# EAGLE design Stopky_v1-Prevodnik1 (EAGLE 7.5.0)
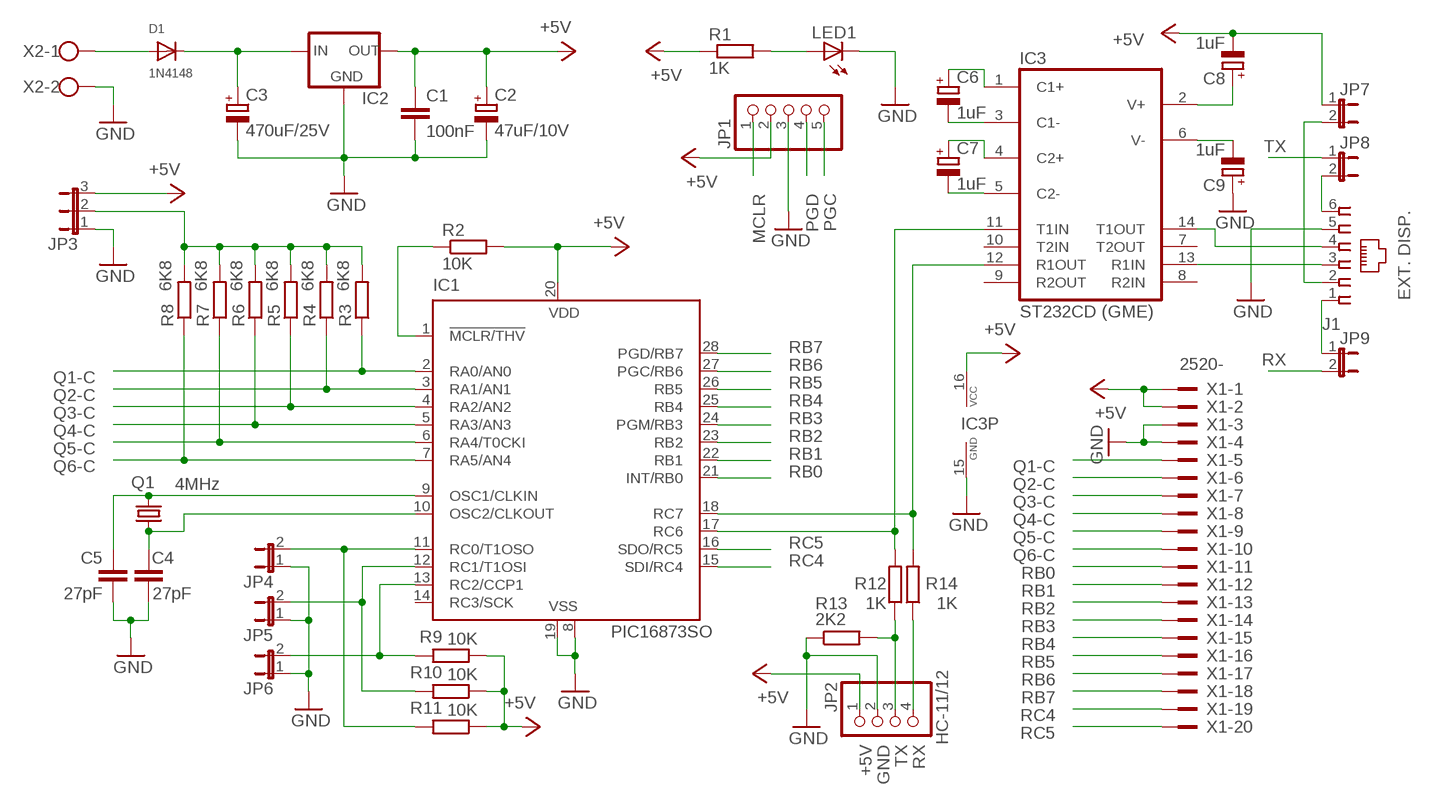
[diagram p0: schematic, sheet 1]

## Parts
C1  100nF  C-EUC1206  [C1206]
C2  47uF/10V  CPOL-EUSMCC  [SMC_C]
C3  470uF/25V  CPOL-EUE3.5-8  [E3,5-8]
C4  27pF  C-EUC1206  [C1206]
C5  27pF  C-EUC1206  [C1206]
C6  1uF  CPOL-EUSMCA  [SMC_A]
C7  1uF  CPOL-EUSMCA  [SMC_A]
C8  1uF  CPOL-EUSMCA  [SMC_A]
C9  1uF  CPOL-EUSMCA  [SMC_A]
D1  1N4148  DIODE_SOD-123FL  [SOD-123FL]
IC1  PIC16873SO  [SO28W]
IC2  78LXX-SOT89  [SOT89]
IC3  ST232CD (GME)  MAX3232CSE  [SO16]
J1  520250-3  [520250-3]
JP1  PINHD-1X5  [1X05]
JP2  PINHD-1X4  [1X04]
JP3  JP2E  [JP2]
JP4  JP1E  [JP1]
JP5  JP1E  [JP1]
JP6  JP1E  [JP1]
JP7  JP1E  [JP1]
JP8  JP1E  [JP1]
JP9  JP1E  [JP1]
LED1  LEDCHIPLED_1206  [CHIPLED_1206]
Q1  4MHz  CRYSTALSM49  [SM49]
R1  1K  R-EU_R1206  [R1206]
R2  10K  R-EU_R1206  [R1206]
R3  6K8  R-EU_R1206  [R1206]
R4  6K8  R-EU_R1206  [R1206]
R5  6K8  R-EU_R1206  [R1206]
R6  6K8  R-EU_R1206  [R1206]
R7  6K8  R-EU_R1206  [R1206]
R8  6K8  R-EU_R1206  [R1206]
R9  10K  R-EU_R1206  [R1206]
R10  10K  R-EU_R1206  [R1206]
R11  10K  R-EU_R1206  [R1206]
R12  1K  R-EU_R1206  [R1206]
R13  2K2  R-EU_R1206  [R1206]
R14  1K  R-EU_R1206  [R1206]
X1  2520-  [PAK100/2500-20]
X2  AK550/2  [AK550/2]

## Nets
+5V: C1.1 C2.+ C8.- IC1.20(VDD) IC2.1(OUT) IC3.16(VCC) JP1.2 JP2.1 JP3.3 JP7.1 R1.1 R2.2 R9.1 R10.1 R11.1 X1.1 X1.2
GND: C1.2 C2.- C3.- C4.2 C5.2 C9.+ IC1.8(VSS) IC1.19(VSS) IC2.2(GND) IC3.15(GND) J1.5 JP1.3 JP2.2 JP3.1 JP4.1 JP5.1 JP6.1 LED1.C R13.1 X1.3 X1.4 X2.2
MCLR: IC1.1(!MCLR/THV) JP1.1 R2.1
N$1: D1.A X2.1
N$2: C3.+ D1.C IC2.3(IN)
N$3: C5.1 IC1.9(OSC1/CLKIN) Q1.2
N$4: C4.1 IC1.10(OSC2/CLKOUT) Q1.1
N$5: LED1.A R1.2
N$6: J1.1 JP9.1
N$8: JP2.3 R12.1 R13.2
N$9: JP2.4 R14.1
N$10: C6.- IC3.3(C1-)
N$11: C7.+ IC3.4(C2+)
N$12: JP3.2 R3.2 R4.2 R5.2 R6.2 R7.2 R8.2
N$13: IC1.11(RC0/T1OSO) JP4.2 R11.2
N$14: IC1.12(RC1/T1OSI) JP5.2 R10.2
N$15: IC1.13(RC2/CCP1) JP6.2 R9.2
N$16: C7.- IC3.5(C2-)
N$17: C6.+ IC3.1(C1+)
N$18: C8.+ IC3.2(V+)
N$19: C9.- IC3.6(V-)
N$20: IC3.13(R1IN) J1.3
N$21: IC3.14(T1OUT) J1.4
N$22: J1.2 JP7.2
N$23: J1.6 JP8.2
PGC: IC1.27(PGC/RB6) JP1.5 X1.17
PGD: IC1.28(PGD/RB7) JP1.4 X1.18
Q1-C: IC1.2(RA0/AN0) R3.1 X1.5
Q2-C: IC1.3(RA1/AN1) R4.1 X1.6
Q3-C: IC1.4(RA2/AN2) R5.1 X1.7
Q4-C: IC1.5(RA3/AN3) R6.1 X1.8
Q5-C: IC1.6(RA4/T0CKI) R7.1 X1.9
Q6-C: IC1.7(RA5/AN4) R8.1 X1.10
RB0: IC1.21(INT/RB0) X1.11
RB1: IC1.22(RB1) X1.12
RB2: IC1.23(RB2) X1.13
RB3: IC1.24(PGM/RB3) X1.14
RB4: IC1.25(RB4) X1.15
RB5: IC1.26(RB5) X1.16
RC4: IC1.15(SDI/RC4) X1.19
RC5: IC1.16(SDO/RC5) X1.20
RX: IC1.18(RC7) IC3.12(R1OUT) JP9.2 R14.2
TX: IC1.17(RC6) IC3.11(T1IN) JP8.1 R12.2
Unconnected: IC1.14(RC3/SCK) IC3.7(T2OUT) IC3.8(R2IN) IC3.9(R2OUT) IC3.10(T2IN)

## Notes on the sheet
- TX
- MCLR | PGD | PGC
- EXT. DISP.
- RB7 | RX
- Q1-C | RB6
- Q2-C | RB5
- Q3-C | RB4
- Q4-C | RB3
- Q5-C | RB2
- Q6-C | RB1 | Q1-C
- RB0 | Q2-C
- Q3-C
- Q4-C
- Q5-C
- RC5 | Q6-C
- RC4 | RB0
- RB1
- RB2
- RB3
- RB4
- RB5
- RB6
- RB7
- RC4
- RC5
- +5V | GND | TX | RX | HC-11/12

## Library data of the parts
C1 C4 C5 = rcl:C-EU: CAPACITOR, European symbol
C2 C3 C6-C9 = rcl:CPOL-EU: POLARIZED CAPACITOR, European symbol
D1 = adafruit:DIODE: Diode
IC1 = microchip-6:PIC16*873: MICROCONTROLLER flash type
IC2 = v-reg-3:78LXX: VOLTAGE REGULATOR
IC3 = maxim:MAX3232*: True RS-232 Transceivers 3.0V to 5.5V, Low-Power up to 1Mbps, Using Four 0.1µF External Capacitors Source: http://pdfserv.maxim-ic.com/en/ds/MAX3222-MAX3241.pdf; MPN: MAX3232CSE; OC_FARNELL: 9725490; OC_NEWARK: 90C2890
J1 = con-amp:520250-3: AMP connector
JP1 = pinhead:PINHD-1X5: PIN HEADER
JP2 = pinhead:PINHD-1X4: PIN HEADER
JP3 = jumper:JP2E: JUMPER
JP4-JP9 = jumper:JP1E: JUMPER
LED1 = adafruit:LED: LED
Q1 = crystal:CRYSTAL: CRYSTAL; OC_FARNELL: unknown; OC_NEWARK: unknown
R1-R14 = rcl:R-EU_: RESISTOR, European symbol
X1 = con-3m:2520-: 3M (TM) Pak 100 4-Wall Header Source: 3M; OC_FARNELL: unknown; OC_NEWARK: unknown
X2 = con-ptr500+:AK550/2: CONNECTOR

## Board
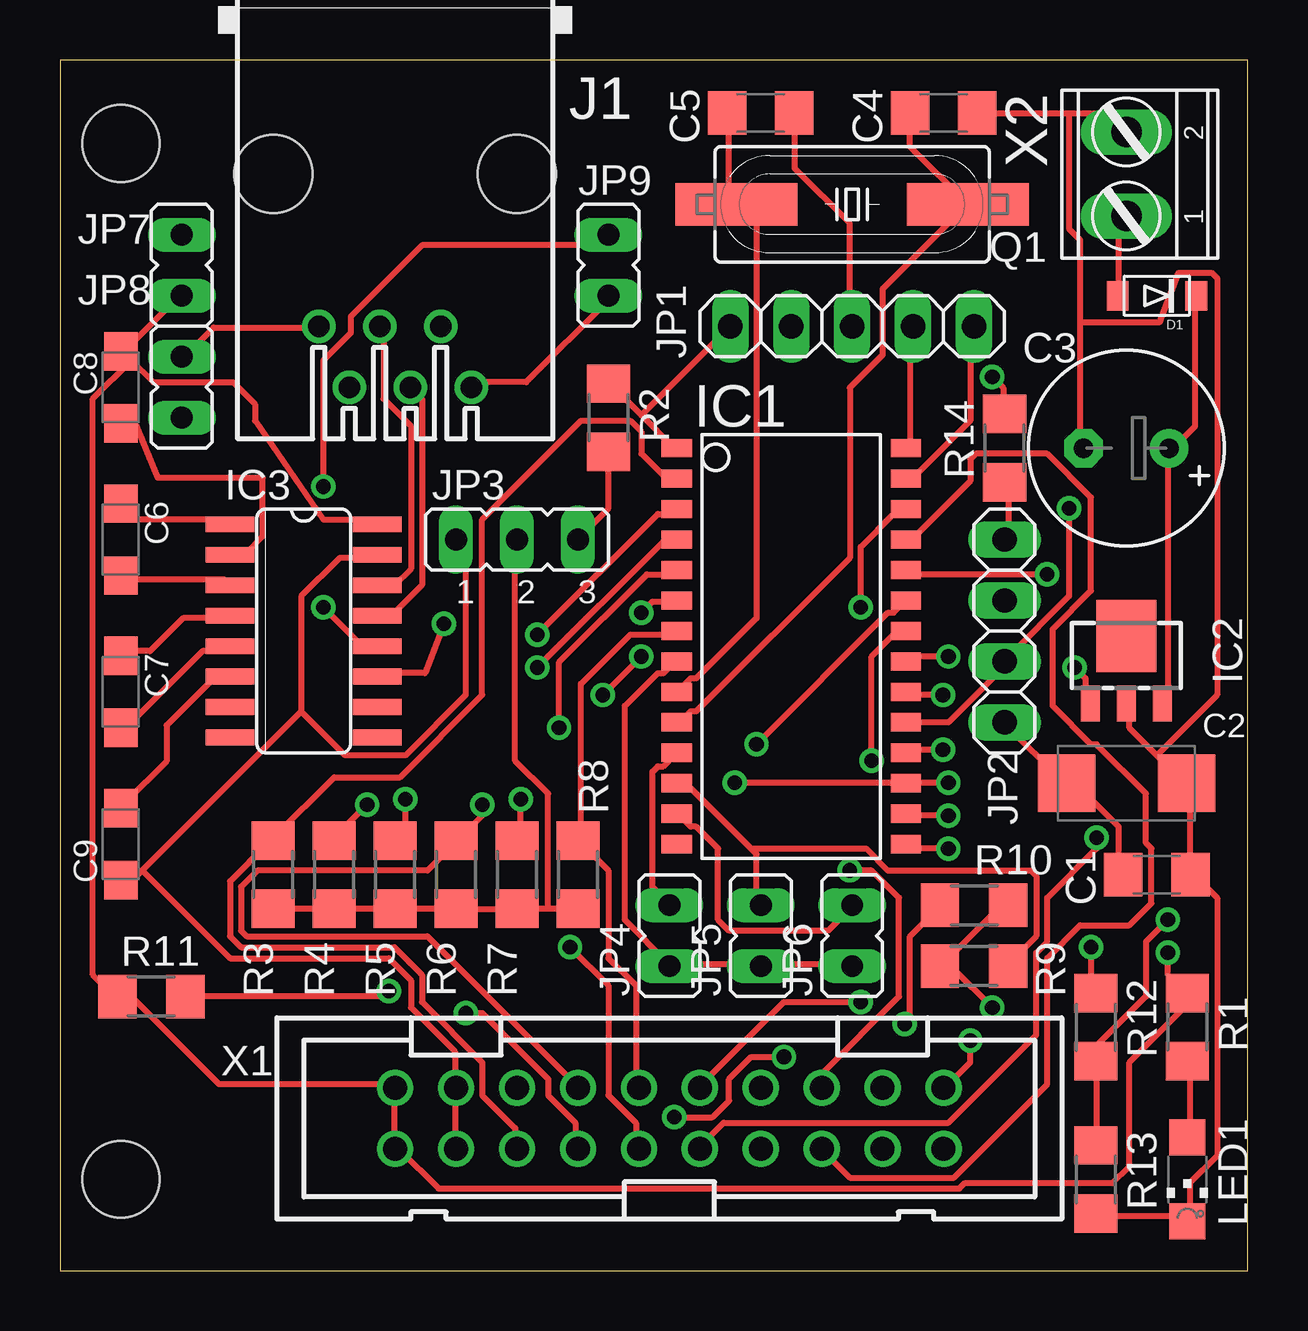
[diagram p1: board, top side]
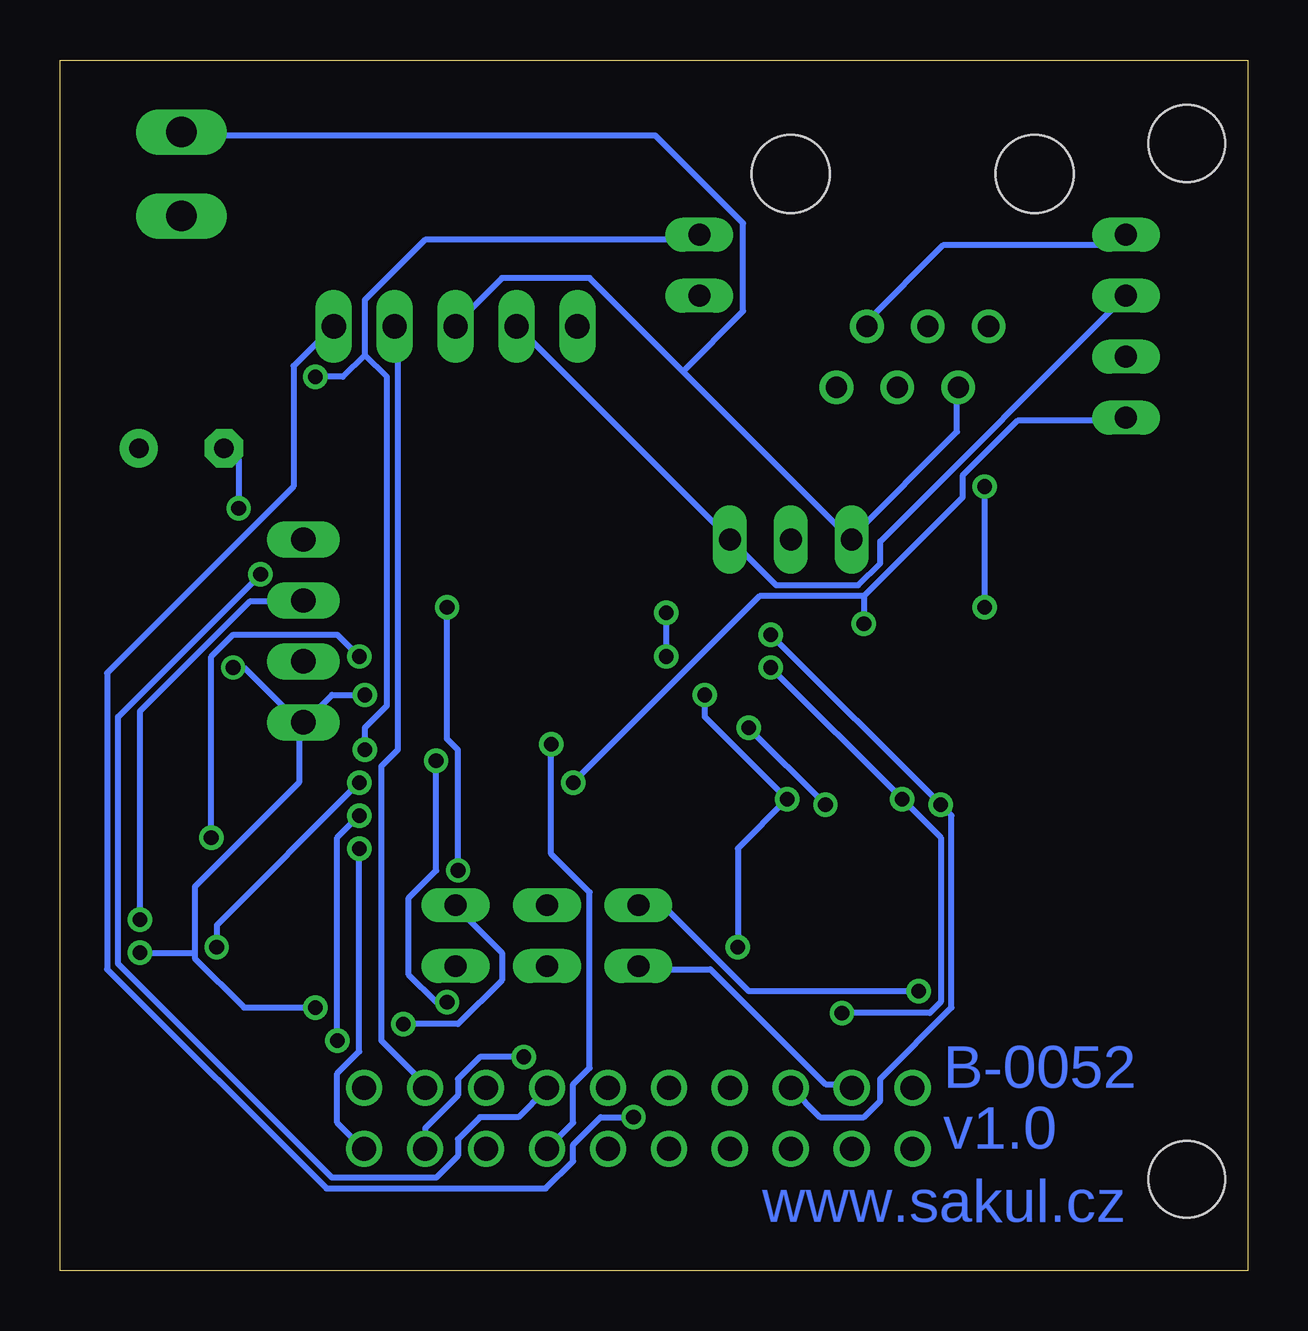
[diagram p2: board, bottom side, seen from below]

Size 49.51 x 50.47 mm. Coordinates in mm from the lower left corner, seen from the top.
Outline: 0,0 49.51,0 49.51,50.47 0,50.47 0,0
Copper layers (1*16): Top 0.035mm / dielectric 1.5mm / Bottom 0.035mm
Design rules "default": minimum track width 10mil, minimum drill 24mil, track to track 8mil, track to pad 8mil, pad to pad 8mil, via to via 8mil, smd to smd 8mil, copper to edge 40mil, drill to drill 8mil, minimum pad ring 10mil, minimum via ring 8mil, stop-mask expansion 4mil, vias tented up to drill 0mil, thermal gap 10mil
Holes 3.2 mm at 2.54,46.99 2.54,3.81

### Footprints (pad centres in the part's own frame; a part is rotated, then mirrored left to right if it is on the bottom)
C1206 = smd 1.6 x 1.8: 1 -1.4,0; 2 1.4,0
SMC_C = smd 2.4 x 2.4: + -2.5,0; - 2.5,0
E3,5-8 = drill 0.813 pad 1.6: + -1.778,0 | drill 0.813 pad 1.6 octagon: - 1.778,0
SMC_A = smd 1.6 x 1.4: + -1.5,0; - 1.5,0
SOD-123FL = smd 0.91 x 1.22: A 1.637,0; C -1.637,0
SO28W = smd 0.762 x 1.27: 1 -7.62,-4.78; 2 -6.35,-4.78; 3 -5.08,-4.78; 4 -3.81,-4.78; 5 -2.54,-4.78; 6 -1.27,-4.78; 7 0,-4.78; 8 1.27,-4.78; 9 2.54,-4.78; 10 3.81,-4.78; 11 5.08,-4.78; 12 6.35,-4.78; 13 7.62,-4.78; 14 8.89,-4.78; 15 8.89,4.78; 16 7.62,4.78; 17 6.35,4.78; 18 5.08,4.78; 19 3.81,4.78; 20 2.54,4.78; 21 1.27,4.78; 22 0,4.78; 23 -1.27,4.78; 24 -2.54,4.78; 25 -3.81,4.78; 26 -5.08,4.78; 27 -6.35,4.78; 28 -7.62,4.78
SOT89 = smd 0.8 x 1.5: 1 -1.5,-1.75; 2 0,-1.75; 3 1.5,-1.75 | smd 2.5 x 3: 4 0,1.05
SO16 = smd 0.66 x 2.032: 1 -4.445,-3.073; 2 -3.175,-3.073; 3 -1.905,-3.073; 4 -0.635,-3.073; 5 0.635,-3.073; 6 1.905,-3.073; 7 3.175,-3.073; 8 4.445,-3.073; 9 4.445,3.073; 10 3.175,3.073; 11 1.905,3.073; 12 0.635,3.073; 13 -0.635,3.073; 14 -1.905,3.073; 15 -3.175,3.073; 16 -4.445,3.073
520250-3 = drill 0.889: 1 -3.175,8.89; 2 -1.905,6.35; 3 -0.635,8.89; 4 0.635,6.35; 5 1.905,8.89; 6 3.175,6.35 | hole 3.251: -5.08,0; 5.08,0
1X05 = drill 1.016 long: 1 -5.08,0; 2 -2.54,0; 3 0,0; 4 2.54,0; 5 5.08,0
1X04 = drill 1.016 long: 1 -3.81,0; 2 -1.27,0; 3 1.27,0; 4 3.81,0
JP2 = drill 0.914 long: 1 -2.54,0; 2 0,0; 3 2.54,0
JP1 = drill 0.914 long: 1 0,-1.27; 2 0,1.27
CHIPLED_1206 = smd 1.5 x 1.5: A 0,-1.75; C 0,1.75
SM49 = smd 5.08 x 1.778: 1 -4.826,0; 2 4.826,0
R1206 = smd 1.6 x 1.803: 1 -1.422,0; 2 1.422,0
PAK100/2500-20 = drill 1 pad 1.422: 1 -11.43,-1.27; 2 -11.43,1.27; 3 -8.89,-1.27; 4 -8.89,1.27; 5 -6.35,-1.27; 6 -6.35,1.27; 7 -3.81,-1.27; 8 -3.81,1.27; 9 -1.27,-1.27; 10 -1.27,1.27; 11 1.27,-1.27; 12 1.27,1.27; 13 3.81,-1.27; 14 3.81,1.27; 15 6.35,-1.27; 16 6.35,1.27; 17 8.89,-1.27; 18 8.89,1.27; 19 11.43,-1.27; 20 11.43,1.27
AK550/2 = drill 1.27 long: 1 -1.75,0; 2 1.75,0

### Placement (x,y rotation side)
C1  45.72,16.51 0 top
C2  44.45,20.32 0 top
C3  44.45,34.29 180 top
C4  36.83,48.26 0 top
C5  29.21,48.26 0 top
C6  2.54,30.48 270 top
C7  2.54,24.13 270 top
C8  2.54,36.83 90 top
C9  2.54,17.78 90 top
D1  45.72,40.64 180 top
IC1  30.48,26.67 270 top
IC2  44.45,25.4 0 top
IC3  10.16,26.67 270 top
J1  13.97,45.72 180 top
JP1  33.02,39.37 0 top
JP2  39.37,26.67 90 top
JP3  19.05,30.48 0 top
JP4  25.4,13.97 0 top
JP5  29.21,13.97 0 top
JP6  33.02,13.97 0 top
JP7  5.08,41.91 0 top
JP8  5.08,36.83 0 top
JP9  22.86,41.91 0 top
LED1  46.99,3.81 180 top
Q1  33.02,44.45 180 top
R1  46.99,10.16 270 top
R2  22.86,35.56 270 top
R3  8.89,16.51 270 top
R4  11.43,16.51 270 top
R5  13.97,16.51 270 top
R6  16.51,16.51 270 top
R7  19.05,16.51 270 top
R8  21.59,16.51 270 top
R9  38.1,15.24 180 top
R10  38.1,12.7 0 top
R11  3.81,11.43 0 top
R12  43.18,10.16 90 top
R13  43.18,3.81 90 top
R14  39.37,34.29 90 top
X1  25.4,6.35 0 top
X2  44.45,45.72 90 top

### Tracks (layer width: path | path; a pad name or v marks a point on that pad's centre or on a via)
+5V  (via drill 0.61)
  Top 0.254: C8.- 2.74,38.41 5.03,40.69 JP7.1 | 2.97,37.95 2.74,38.18 C8.- | 2.97,37.95 3.89,37.03 7.21,37.03 8.13,36.12 8.13,35.43 10.97,31.32 13.03,31.32 IC3.16 | R2.2 22.86,31.77 21.72,30.63 JP3.3 | C1.1 44.12,16.69 44.12,18.52 42.52,20.12 42.06,20.12 C2.+ 41.83,20.34 39.32,22.86 JP2.1 | R9.1 39.32,15.32 36.8,12.8 R10.1 36.8,12.57 37.26,12.57 v38.86,10.97 | v36.8,24 35.43,24 IC1.20 | v42.29,25.15 42.75,24.69 42.75,23.77 IC2.1 | v46.18,13.26 46.18,12.34 46.86,11.66 R1.1 46.86,11.43 46.86,10.97 44.58,8.69 44.58,4.34 43.89,3.66 37.72,3.66 37.49,3.43 15.77,3.43 14.17,5.03 X1.1 13.95,5.26 13.95,7.54 X1.2 13.95,7.77 6.63,7.77 2.97,11.43 R11.1 2.29,11.43 1.37,12.34 1.37,36.35 2.97,37.95 | 2.97,37.95 C8.-
  Bottom 0.254: JP1.2 30.4,39.32 21.72,30.63 JP3.3 21.49,30.4 19.66,28.57 16.23,28.57 15.32,29.49 15.32,30.4 JP7.1 | v36.8,24 38.18,24 39.32,22.86 JP2.1 39.55,22.86 | v42.29,25.15 41.83,25.15 39.55,22.86 | v38.86,10.97 41.83,10.97 43.89,13.03 43.89,13.26 | 43.89,13.26 43.89,16 39.55,20.34 39.55,22.86 | v46.18,13.26 43.89,13.26
GND  (via drill 0.61)
  Top 0.254: R13.1 43.2,2.29 46.86,2.29 LED1.C 47.09,2.29 47.09,3.66 48.23,4.8 48.23,15.54 47.32,16.46 C1.2 47.09,16.69 47.09,20.12 C2.- 46.86,20.34 45.72,21.49 | 45.72,21.49 44.58,22.63 44.58,23.55 IC2.2 | IC1.19 37.03,22.86 39.55,25.38 JP2.2 39.55,25.6 42.06,28.12 v42.06,31.77 | 42.06,48.23 43.66,48.23 44.35,47.55 X2.2 | 42.06,48.23 38.41,48.23 C4.2 | 42.52,39.55 42.52,42.98 42.06,43.43 42.06,48.23 | 42.52,39.55 42.52,34.29 C3.- | 45.72,21.49 48.23,24 48.23,41.38 48.01,41.6 46.63,41.6 45.85,39.55 42.52,39.55 | X1.3 16.46,5.26 16.46,7.54 X1.4 16.46,7.77 16.46,9.14 14.63,10.97 14.63,12.12 13.72,13.03 7.09,13.03 3.43,16.69 | IC1.8 25.6,25.38 25.15,24.92 24.92,24.92 23.55,23.55 23.55,14.63 25.38,12.8 JP4.1 25.6,12.8 29.03,12.8 JP5.1 29.26,12.8 32.92,12.8 JP6.1 | 10.06,23.32 3.43,16.69 | 3.43,16.69 3.2,16.46 2.74,16.46 C9.+ | 10.06,23.32 10.06,28.12 11.66,29.72 13.03,29.72 IC3.15 | C5.2 30.63,48.23 30.63,45.95 32.92,43.66 32.92,39.55 JP1.3 | 10.06,23.32 11.89,21.49 14.4,21.49 16.92,24 16.92,30.18 16.69,30.4 JP3.1
  Bottom 0.254: v42.06,31.77 42.06,33.83 42.52,34.29 C3.- | X1.4 16.69,7.77 17.6,7.77 22.4,12.57 25.38,12.57 JP4.1 | J1.5 12.12,36.8 12.12,34.98 16.46,30.63 JP3.1 16.69,30.63 23.55,37.49 | 23.55,37.49 27.43,41.38 31.09,41.38 32.92,39.55 JP1.3 | 23.55,37.49 21.03,40.01 21.03,43.66 24.69,47.32 44.35,47.32 X2.2
MCLR
  Top 0.254: 24.23,35.66 22.86,37.03 R2.1 | 24.23,35.66 25.6,34.29 IC1.1 | 24.23,35.66 JP1.1
N$1
  Top 0.254: D1.A 44.12,40.69 44.12,43.66 44.35,43.89 X2.1
N$2
  Top 0.254: D1.C 47.32,40.46 47.32,35.2 46.41,34.29 C3.+ 46.18,34.29 46.18,23.77 IC2.3
N$3
  Top 0.254: IC1.9 25.83,24.23 26.29,24.69 26.52,24.69 29.03,27.2 29.03,43.66 28.35,44.35 Q1.2 28.12,44.58 27.89,44.81 27.89,48.23 C5.1
N$4
  Top 0.254: IC1.10 25.83,22.86 26.29,23.32 26.52,23.32 32.92,29.72 32.92,36.8 34.29,38.18 34.29,40.92 37.72,44.35 Q1.1 35.43,46.86 35.43,48.23 C4.1
N$5
  Top 0.254: LED1.A 47.09,5.71 47.09,8.69 R1.2
N$6
  Top 0.254: J1.1 17.14,37.03 19.43,37.03 22.86,40.46 JP9.1
N$8  (via drill 0.61)
  Top 0.254: R13.2 43.2,5.26 43.2,8.69 R12.1 43.2,8.91 43.2,9.37 45.26,11.43 45.26,13.72 v46.18,14.63
  Bottom 0.254: v46.18,14.63 46.18,23.32 41.6,27.89 39.55,27.89 JP2.3
N$9
  Top 0.254: R14.1 39.55,32.69 39.55,30.63 JP2.4
N$10
  Top 0.254: IC3.3 6.86,28.8 2.74,28.8 C6.-
N$11
  Top 0.254: C7.+ 2.74,25.83 3.76,25.83 5.13,27.2 7.09,27.2 IC3.4
N$12
  Top 0.254: 20.34,15.09 21.49,15.09 R8.2 | 20.34,15.09 19.2,15.09 R7.2 18.97,15.09 16.69,15.09 R6.2 16.46,15.09 14.17,15.09 R5.2 13.95,15.09 R4.2 | R4.2 8.91,15.09 R3.2 | R4.2 | 20.34,15.09 20.34,19.89 18.97,21.26 18.97,30.4 JP3.2
N$13  (via drill 0.61)
  Top 0.254: IC1.11 25.6,21.49 25.15,21.03 24.92,21.03 24.69,20.8 24.69,16 25.38,15.32 JP4.2 | R11.2 13.49,11.43 v13.72,11.66
  Bottom 0.254: v13.72,11.66 20.8,11.66 24.23,15.09 25.38,15.09 JP4.2
N$14
  Top 0.254: 28.8,17.6 29.03,17.37 29.03,15.32 JP5.2 | 28.8,17.6 26.29,20.12 25.83,20.12 IC1.12 | 28.8,17.6 33.6,17.6 34.52,16.69 40.46,16.69 40.69,16.46 40.69,13.95 39.55,12.8 R10.2
N$15  (via drill 0.61)
  Top 0.254: IC1.13 25.83,18.97 26.29,18.52 26.52,18.52 27.43,17.6 27.43,14.63 27.89,14.17 32,14.17 32.92,15.09 JP6.2 | v35.2,10.29 35.43,10.52 35.43,13.95 36.58,15.09 R9.2
  Bottom 0.254: v35.2,10.29 32.92,10.29 31.09,12.12 31.09,13.26 32.92,15.09 JP6.2
N$16
  Top 0.254: C7.- 2.74,22.63 5.94,25.83 7.09,25.83 IC3.5
N$17
  Top 0.254: C6.+ 2.74,31.77 2.13,31.77 2.59,31.32 7.09,31.32 IC3.1
N$18
  Top 0.254: C8.+ 2.74,35.2 3.2,35.2 4.09,33.05 8.46,33.05 8.46,30.63 7.77,29.95 7.09,29.95 IC3.2
N$19
  Top 0.254: C9.- 2.74,19.43 2.74,19.53 4.45,21.23 4.45,22.73 6.4,24.69 7.09,24.69 IC3.6
N$20
  Top 0.254: J1.3 15.09,36.35 15.09,28.57 13.95,27.43 13.26,27.43 IC3.13
N$21
  Top 0.254: IC3.14 13.95,28.57 14.63,29.26 14.63,35.2 13.49,36.35 13.49,39.32 J1.4
N$22
  Bottom 0.254: J1.2 15.77,39.55 15.9,39.55 12.7,42.75 5.49,42.75 5.26,42.98 JP7.2
N$23
  Top 0.254: J1.6 10.74,39.32 6.4,39.32 5.26,38.18 JP8.2
PGC  (via drill 0.61)
  Top 0.254: IC1.27 35.43,33.15 35.66,33.15 37.95,35.43 37.95,39.32 JP1.5 | v30.18,8.91 28.8,8.91 27.89,8 27.89,7.09 27.2,6.4 v25.6,6.4
  Bottom 0.254: X1.17 34.29,5.94 32.92,7.32 32.92,8 32,8.91 v30.18,8.91 | v25.6,6.4 26.98,6.4 28.12,5.26 28.12,4.57 29.26,3.43 38.41,3.43 47.55,12.57 47.55,24.92 39.78,32.69 39.78,37.72 38.18,39.32 JP1.5
PGD
  Top 0.254: IC1.28 35.43,34.29 35.43,39.32 JP1.4
  Bottom 0.254: X1.18 34.29,7.77 36.12,9.6 36.12,21.03 35.43,21.72 35.43,39.32 JP1.4
Q1-C
  Top 0.254: IC1.2 25.6,33.15 25.15,33.15 24.23,34.06 24.23,34.98 23.77,35.43 21.72,35.43 17.6,31.32 17.6,24 14.17,20.57 11.43,20.57 8.91,18.06 R3.1 8.69,17.83 7.09,16.23 7.09,13.95 7.54,13.49 13.95,13.49 15.09,12.34 15.09,11.2 17.6,8.69 17.6,7.32 18.97,5.94 18.97,5.26 X1.5
Q2-C  (via drill 0.61)
  Top 0.254: v19.89,26.52 24.92,31.55 25.6,31.55 IC1.3 | v12.8,19.43 11.43,18.06 R4.1
  Bottom 0.254: v19.89,26.52 v12.8,19.43 12.34,18.97 12.34,10.97 15.32,8 15.32,7.09 16,6.4 17.83,6.4 X1.6
Q3-C  (via drill 0.61)
  Top 0.254: v19.89,25.15 25.15,30.4 25.6,30.4 IC1.4 | v14.4,19.66 14.4,18.29 14.17,18.06 R5.1 | v16.92,10.74 17.6,10.74 20.34,8 20.34,7.32 21.49,6.17 21.49,5.26 X1.7
  Bottom 0.254: v19.89,25.15 v14.4,19.66 12.8,18.06 12.8,11.2 13.26,10.74 v16.92,10.74
Q4-C  (via drill 0.61)
  Top 0.254: v20.8,22.63 20.8,25.38 24.46,29.03 25.6,29.03 IC1.5 | v17.6,19.43 17.6,18.97 16.69,18.06 R6.1 16.46,17.83 15.32,16.69 8.23,16.69 7.54,16 7.54,14.17 7.77,13.95 15.32,13.95 21.49,7.77 X1.8
  Bottom 0.254: v17.6,19.43 v20.8,22.63
Q5-C  (via drill 0.61)
  Top 0.254: v24.23,27.43 24.69,27.89 25.6,27.89 IC1.6 | v22.63,24 v24.23,25.6 | v19.2,19.66 19.2,18.06 R7.1 | v21.26,13.49 22.86,11.89 22.86,7.32 24,6.17 24,5.26 X1.9
  Bottom 0.254: v24.23,25.6 v24.23,27.43 | v22.63,24 22.63,23.09 v19.2,19.66 21.26,17.6 v21.26,13.49
Q6-C
  Top 0.254: IC1.7 25.6,26.52 23.77,26.52 21.72,24.46 21.72,18.06 R8.1 21.72,17.83 22.86,16.69 22.86,13.03 24,11.89 24,7.77 X1.10
RB0  (via drill 0.61)
  Top 0.254: v37.03,25.6 35.43,25.6 IC1.21 | v43.2,18.06 43.2,17.6 41.15,15.54 41.15,13.72 40.69,13.26 40.69,9.83 37.03,6.17 27.66,6.17 26.75,5.26 X1.11
  Bottom 0.254: v37.03,25.6 37.95,26.52 42.29,26.52 43.2,25.6 v43.2,18.06
RB1  (via drill 0.61)
  Top 0.254: v33.83,21.26 33.83,25.6 34.75,26.52 35.2,26.52 IC1.22 | v33.38,11.2 30.18,11.2 26.75,7.77 X1.12
  Bottom 0.254: v33.83,21.26 33.83,16.69 34.98,15.54 34.98,12.34 33.83,11.2 v33.38,11.2
RB2  (via drill 0.61)
  Top 0.254: v29.03,21.95 34.52,27.43 34.75,27.43 35.2,27.89 IC1.23
  Bottom 0.254: v29.03,21.95 29.03,17.37 27.43,15.77 27.43,8.46 28.12,7.77 28.12,6.17 X1.13
RB3  (via drill 0.61)
  Top 0.254: v41.15,29.03 35.43,29.03 IC1.24
  Bottom 0.254: v41.15,29.03 47.09,23.09 47.09,12.8 38.18,3.89 33.83,3.89 32.92,4.8 32.92,5.49 32,6.4 30.4,6.4 29.26,7.54 X1.14
RB4
  Top 0.254: IC1.25 35.43,30.63 35.66,30.63 37.95,32.92 37.95,33.83 38.18,34.06 41.15,34.06 42.98,32.23 42.98,28.35 41.38,26.75 41.38,23.55 42.98,21.95 43.2,21.95 45.26,19.89 45.26,17.83 45.49,17.6 45.49,15.32 44.58,14.4 42.52,14.4 41.15,13.03 41.15,7.77 37.26,3.89 32.92,3.89 31.77,5.03 X1.15
RB5  (via drill 0.61)
  Top 0.254: v33.38,27.66 33.38,30.18 34.75,31.55 35.2,31.55 IC1.26 | v32.92,16.69 33.83,16.69 34.98,15.54 34.98,11.43 31.77,8.23 31.77,7.77 X1.16
  Bottom 0.254: v33.38,27.66 33.38,22.17 32.92,21.72 v32.92,16.69
RC4  (via drill 0.61)
  Top 0.254: v37.03,17.6 35.43,17.6 IC1.15
  Bottom 0.254: v37.03,17.6 37.03,9.14 37.95,8.23 37.95,6.17 37.03,5.26 X1.19
RC5  (via drill 0.61)
  Top 0.254: v37.03,18.97 35.43,18.97 IC1.16 | v37.95,9.6 37.95,8.69 37.03,7.77 X1.20
  Bottom 0.254: v37.03,18.97 37.95,18.06 v37.95,9.6
RX  (via drill 0.61)
  Top 0.254: v36.8,21.72 35.43,21.72 IC1.18 | v38.86,37.26 39.32,36.8 39.32,35.89 R14.2 | v10.97,27.66 12.57,26.06 13.03,26.06 IC3.12 | v10.97,32.69 10.97,37.95 12.12,39.09 12.12,39.78 15.09,42.75 22.63,42.75 22.86,42.98 JP9.2
  Bottom 0.254: v36.8,21.72 36.8,22.63 35.89,23.55 35.89,37.26 36.8,38.18 | 36.8,38.18 36.8,40.46 34.29,42.98 22.86,42.98 JP9.2 | v38.86,37.26 37.72,37.26 36.8,38.18 | v10.97,32.69 v10.97,27.66
TX  (via drill 0.61)
  Top 0.254: v28.12,20.34 35.2,20.34 IC1.17 35.43,20.34 v37.03,20.34 | v42.98,13.49 42.98,11.66 R12.2 | v16,26.98 15.21,24.92 13.26,24.92 IC3.11
  Bottom 0.254: v28.12,20.34 20.34,28.12 16,28.12 | 16,28.12 11.89,32.23 11.89,33.15 9.6,35.43 5.26,35.43 JP8.1 | v42.98,13.49 42.98,14.4 v37.03,20.34 | 16,28.12 v16,26.98

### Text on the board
Bottom: B-0052 | v1.0 | www.sakul.cz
